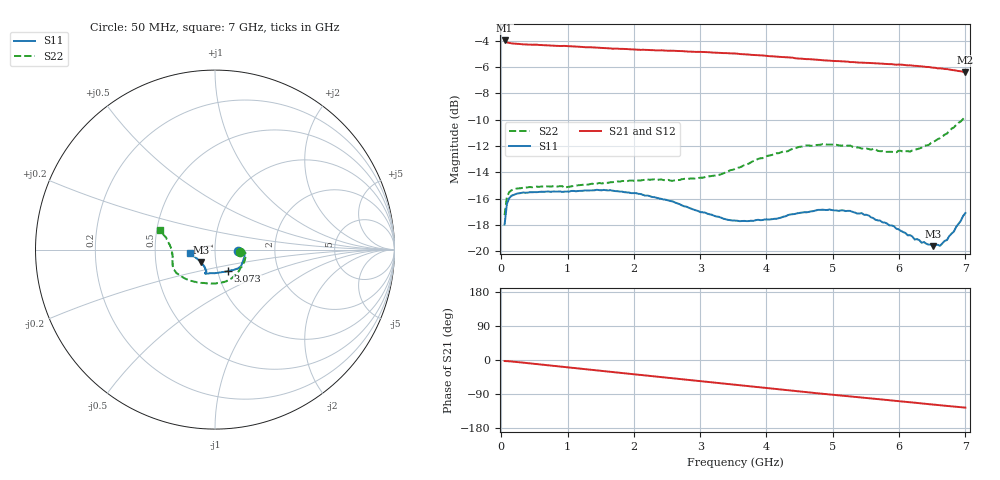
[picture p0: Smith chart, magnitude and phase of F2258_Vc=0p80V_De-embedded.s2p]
! Integrated Device Technology
! Corporate Headquarters
! 6024 Silver Creek Valley Road
! San Jose, CA 95138  USA
! Phone:  1-408-284-8200
! Toll Free:  1-800-223-1366
! Webpage:  http://www.idt.com/
! Timing and RF Division
! 515 Groton Road, Suite 102
! Westford, MA 01886-6024
! Device:  F2258
! Description: Voltage Variable RF Attenuator
! Frequency:  50.0 -  6000.00 MHz
! Package:  3x3 mm Thin QFN Plastic Package: 16 pin
! Ports:  2 RF, 2 DC
!  Pin  1  = NC
!  Pin  2  = NC
!  Pin  3  = RF2  = Port 2
!  Pin  4  = GND
!  Pin  5  = Vdd
!  Pin  6  = NC
!  Pin  7  = VCTRL
!  Pin  8  = NC
!  Pin  9  = GND
!  Pin 10  = RF1  = Port 1
!  Pin 11  = NC
!  Pin 12  = NC
!  Pin 13  = NC
!  Pin 14  = NC
!  Pin 15  = NC
!  Pin 16  = NC
! Vcntrl:  0.800 Volts
! Vdd:  +3.300 Volts
! Current:  1.132 mA
! Data:  The device was measured on a the F2258 evaluation board which has
!  individual transmission lines to the RF pins.  Data was collected
!  using a calibrated network analyzer.  The evaluation board was
!  de-embedded using a TRL calibration technique.
!  The reference plane is the edge of the package pin.
! Misc:  SN 10
!  Action Tracker AT0285
! Date Measured:  2014-12-10
! Date:  2016-01-13  MJV
! Note:
!  Integrated Device Technology supplies this data as a sample of measured
!  data at the package pin for this product.  Your particular data for this
!  product may vary.
!  Data was taken at 25 degrees C.
!  Integrated Device Technology reserves the right to change this data at anytime.
!Freq_(GHz)  S11M_(dB)  S11P_(deg)  S21M_(dB)  S21P_(deg)  S12M_(dB)  S12P_(deg)  S22M_(dB)  S22P_(deg)
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# GHz S dB R 50
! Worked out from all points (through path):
!   201 points, 50 MHz to 7 GHz, reference 50 ohm
!   highest |S21| = -3.97 dB at 50 MHz (marker M1); lowest = -6.4 dB at 7 GHz (marker M2)
!   group delay of S21, straight-line fit = 49.7 ps
!   lowest |S11| = -19.6 dB at 6.513 GHz (marker M3), VSWR 1.23, Z = 42.5 - j6.1 ohm
!   |S11| at or under -10 dB: start of sweep to end of sweep
!   |S22| runs from -17.2 to -9.8 dB; largest |S21 - S12| = 0.0026
!   S11 on the Smith chart (normalised r, x): 50 MHz: 1.29, -0.03; 3.073 GHz: 1.12, -0.28; 7 GHz: 0.76, -0.03
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0.05  -17.96 -4.4  -3.97 -2.7  -3.98 -2.7  -17.24 -4.7
0.08475  -16.39 -3.4  -4.11 -2.9  -4.12 -2.9  -15.85 -4.3
0.15425  -15.77 -4.0  -4.19 -3.9  -4.20 -3.9  -15.35 -6.4
0.6755  -15.46 -15.6  -4.33 -13.5  -4.35 -13.5  -15.06 -24.2
0.9535  -15.46 -22.6  -4.38 -18.7  -4.39 -18.7  -15.17 -34.6
1.2315  -15.39 -27.5  -4.47 -23.8  -4.48 -23.8  -14.94 -43.6
1.6485  -15.35 -33.7  -4.57 -31.3  -4.58 -31.3  -14.74 -55.7
2.37825  -15.98 -43.1  -4.72 -44.3  -4.72 -44.3  -14.55 -75.6
2.58675  -16.20 -47.0  -4.75 -48.1  -4.75 -48.1  -14.64 -81.9
3.07325  -17.06 -59.1  -4.85 -57.0  -4.87 -57.0  -14.35 -99.4
3.525  -17.66 -76.0  -4.96 -65.5  -4.97 -65.5  -13.74 -117.3
4.11575  -17.53 -98.9  -5.19 -76.3  -5.19 -76.3  -12.60 -137.6
4.7065  -16.94 -110.4  -5.42 -86.7  -5.40 -86.7  -11.97 -151.5
5.2625  -16.92 -112.8  -5.61 -96.2  -5.59 -96.1  -11.96 -160.7
5.5405  -17.27 -112.4  -5.68 -100.9  -5.66 -100.9  -12.21 -165.4
5.85325  -18.03 -113.7  -5.77 -106.1  -5.74 -106.2  -12.43 -172.0
6.166  -18.77 -119.4  -5.86 -111.5  -5.87 -111.5  -12.42 -179.0
6.2355  -19.10 -122.0  -5.90 -112.7  -5.89 -112.7  -12.27 178.9
6.5135  -19.60 -137.2  -6.04 -117.6  -6.04 -117.6  -11.68 171.7
6.61775  -19.58 -144.8  -6.09 -119.3  -6.11 -119.3  -11.40 168.9
6.722  -19.14 -152.6  -6.14 -121.2  -6.16 -121.2  -11.05 166.1
7  -17.09 -171.3  -6.38 -125.7  -6.38 -125.7  -9.75 160.4
